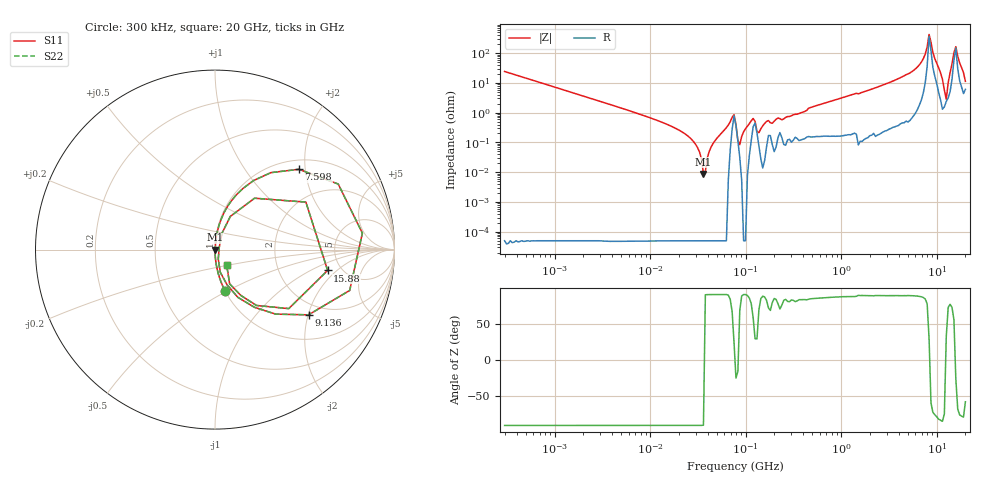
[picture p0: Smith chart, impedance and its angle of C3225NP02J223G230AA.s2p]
! S-Parameter Data Generated by TDK Corporation
! Copyright(C) 2025 TDK Corporation.
! All Rights Reserved.
! TDK P/N: C3225NP02J223G230AA (Multilayer Ceramic Chip Capacitor)
! Property: C=22nF
! Size(LxWxT): 3.2x2.5x2.3mm
! Model Type: s2p (Touchstone File Format Version 1.0)
! Frequency: DC=Yes Start=0.3MHz Stop=20000MHz 243points Log-sweep
! Model Generated on July 30, 2025
! Terms and conditions regarding TDK Simulation Models:
! 1)This simulation model is being provided solely for informational
!  purposes. Please refer to the specifications of the products in
!  terms of detailed characteristics of such products.
! 2)In no event shall TDK Corporation of any of its subsidiaries be
!  liable for any loss or damage arising, directly or indirectly,
!  from any information contained in this simulation model, including,
!  but not limited to loss or damages arising from any inaccuracies,
!  omissions or errors in connection with such information.
! 3)Any and all copyrights on this simulation model are owned by
!  TDK Corporation.  Duplication or redistribution of this simulation
!  model without prior written permission from TDK Corporation
!  is prohibited.
! 4)This simulation model is subject to any modification or change
!  without any prior notice.
! 5)Neither TDK Corporation nor any of its subsidiaries shall make any
!  warranty, express or implied, including but not limited to the
!  correctness, implied warranties of merchantability and fitness for
!  a particular purpose with respect to this simulation models.
! 6)The use of this simulation model shall be deemed to have consented
!  to the terms and conditions hereof.
! Port Assignments:
!  1 ---| |--- 2
! Applicable Conditions:
!  Temperature = 25 degC
!  DC Bias Voltage = 0 V
!  Small Signal Operation
# Hz S MA R 50
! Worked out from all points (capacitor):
!   242 points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, 300 kHz to 20 GHz, reference 50 ohm
!   read as one part in series: C = 21.9 nF near 314.2 kHz
!   lowest |Z| = 8.74 mohm at 36.21 MHz (marker M1)
!   series resonance near 36.98 MHz, so ESL is about 850 pH
!   S11 on the Smith chart (normalised r, x): 300 kHz: 1.00, -0.48; 7.598 GHz: 1.20, +1.85; 9.136 GHz: 1.65, -2.01; 15.88 GHz: 3.89, -1.52; 20 GHz: 1.12, -0.19
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300000  0.2351 -76.4  0.972 13.6  0.972 13.6  0.2351 -76.4
1985118  0.03643 -87.9  0.9993 2.1  0.9993 2.1  0.03643 -87.9
1.254397e7  0.005154 -91.5  0.9998 0.3  0.9998 0.3  0.005154 -91.5
2.622373e7  0.001435 -97.4  0.9998 0.1  0.9998 0.1  0.001435 -97.4
3.620829e7  0.0002119 -155.8  0.9998 0.0  0.9998 0.0  0.0002119 -155.8
7.569506e7  0.008455 23.1  0.9922 -0.2  0.9922 -0.2  0.008455 23.1
7.926541e7  0.00407 -25.9  0.9963 0.1  0.9963 0.1  0.00407 -25.9
8.691929e7  0.0008409 68.1  0.9997 -0.0  0.9997 -0.0  0.0008409 68.1
1.200134e8  0.006386 57.8  0.9966 -0.3  0.9966 -0.3  0.006386 57.8
1.378092e8  0.002143 68.9  0.9992 -0.1  0.9992 -0.1  0.002143 68.9
1.657079e8  0.005091 81.7  0.9993 -0.3  0.9993 -0.3  0.005091 81.7
5.008786e8  0.01566 83.5  0.9984 -0.9  0.9984 -0.9  0.01566 83.5
3.165055e9  0.1009 82.6  0.9921 -5.8  0.9921 -5.8  0.1009 82.6
6.034042e9  0.2852 71.5  0.9491 -16.6  0.9491 -16.6  0.2852 71.5
7.597827e9  0.6469 43.8  0.6947 -40.0  0.6947 -40.0  0.6469 43.8
8.331474e9  0.8263 6.4  0.1949 -23.5  0.1949 -23.5  0.8263 6.4
9.135962e9  0.6353 -34.9  0.5995 37.2  0.5995 37.2  0.6353 -34.9
1.098548e10  0.207 -71.1  0.9526 11.8  0.9526 11.8  0.207 -71.1
1.261444e10  0.02625 26.6  0.9767 -1.0  0.9767 -1.0  0.02625 26.6
1.516815e10  0.5714 27.6  0.558 -27.8  0.558 -27.8  0.5714 27.6
1.58836e10  0.6381 -10.5  0.3873 15.9  0.3873 15.9  0.6381 -10.5
2e10  0.1058 -52.3  0.9391 5.1  0.9391 5.1  0.1058 -52.3
